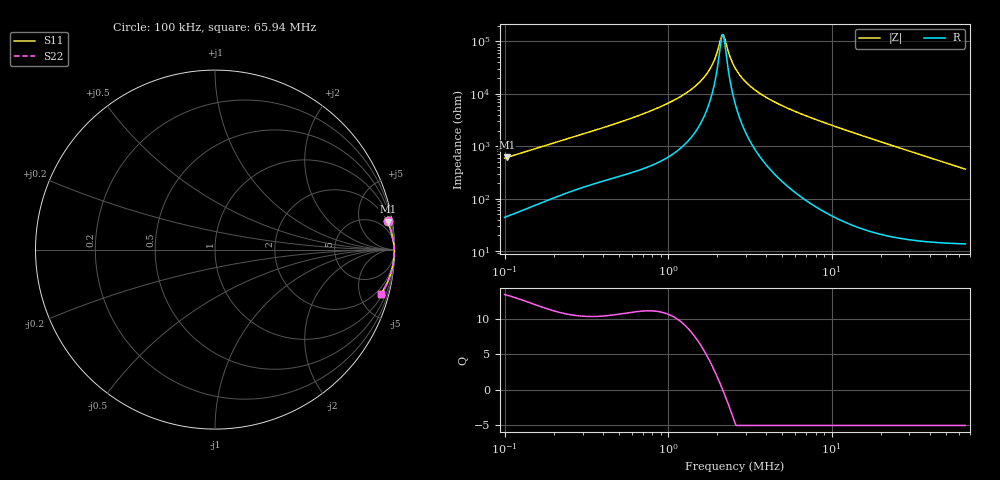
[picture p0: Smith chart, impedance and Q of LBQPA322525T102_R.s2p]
! LBQPA322525T102_R  S-PARAMETER MODEL  ( General Type )
! Model Generated by TAIYO YUDEN Corporation (http://www.ty-top.com)
! Version 1.0
! TAIYO YUDEN Control No. 191025NI43SB-FBB
! Copyright(c) 2019 TAIYO YUDEN CO.,LTD. All Rights Reserved.
! Product Description (link to TY-COMPAS)
! https://ds.yuden.co.jp/TYCOMPAS/or/detail?pn=LBQPA322525T102KR&u=M
! Products Name : Inductors
! Characteristics :
!  Inductance : 1000 uH , SRF(min) : 1.6 MHz , DC Resistance(max) : 16.9 Ohm
!  Rated Current : Saturation :100 mA , Temp Rise : 75 mA (20 degC)
!  Case Size : 3.2 x 2.5 / 0.126 x 0.098 [mm/inch] , Thickness : 2.5 / 0.098 [mm/inch]
!  (Conditions: Temperature = 25 degC , DC Bias Current/Voltage = 0A / 0V)
! External Node Assignments :
!  1  o---GGG---o  2
! GND o---------o GND
! Frequency Range : 0.1MHz  -  65.935307MHz  [ 402 STEP ]
# MHz S RI R 50
! Freq[MHz].  S11 Real  S11 Imag  S21 Real  S21 Imag  S12 Real  S12 Imag  S22 Real  S22 Imag
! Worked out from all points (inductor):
!   401 points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, 100 kHz to 65.94 MHz, reference 50 ohm
!   read as one part in series: L = 932 uH near 103.3 kHz
!   highest Q = 13.3 at 103.3 kHz (marker M1), where L = 941 uH
!   self-resonance near 2.148 MHz
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0.1  0.9612 0.1595  0.0388 -0.1595  0.0388 -0.1595  0.9612 0.1595
0.103299  0.963 0.1549  0.037 -0.1549  0.037 -0.1549  0.963 0.1549
0.296621  0.9909 0.0581  0.00906 -0.0581  0.00906 -0.0581  0.9909 0.0581
0.567694  0.9963 0.0304  0.00374 -0.0304  0.00374 -0.0304  0.9963 0.0304
0.879842  0.998 0.018  0.00196 -0.018  0.00196 -0.018  0.998 0.018
1.25735  0.9988 0.0101  0.0012 -0.0101  0.0012 -0.0101  0.9988 0.0101
1.431655  0.999 0.00753  0.00103 -0.00753  0.00103 -0.00753  0.999 0.00753
1.603884  0.9991 0.00539  0.000912 -0.00539  0.000912 -0.00539  0.9991 0.00539
1.73945  0.9992 0.0039  0.000846 -0.0039  0.000846 -0.0039  0.9992 0.0039
1.856107  0.9992 0.00272  0.000801 -0.00272  0.000801 -0.00272  0.9992 0.00272
1.948707  0.9992 0.00185  0.000773 -0.00185  0.000773 -0.00185  0.9992 0.00185
2.113418  0.9993 0.000397  0.000734 -0.000397  0.000734 -0.000397  0.9993 0.000397
2.147995  0.9993 0.000107  0.000727 -0.000107  0.000727 -0.000107  0.9993 0.000107
2.218855  0.9993 -0.000473  0.000715 0.000473  0.000715 0.000473  0.9993 -0.000473
2.4064  0.9993 -0.00193  0.000691 0.00193  0.000691 0.00193  0.9993 -0.00193
2.609798  0.9993 -0.00339  0.000676 0.00339  0.000676 0.00339  0.9993 -0.00339
3.020209  0.9993 -0.0061  0.000671 0.0061  0.000671 0.0061  0.9993 -0.0061
3.729566  0.9993 -0.0103  0.000713 0.0103  0.000713 0.0103  0.9993 -0.0103
4.994806  0.9991 -0.0168  0.000884 0.0168  0.000884 0.0168  0.9991 -0.0168
7.616602  0.9985 -0.029  0.0015 0.029  0.0015 0.029  0.9985 -0.029
22.59246  0.9898 -0.0918  0.0102 0.0918  0.0102 0.0918  0.9898 -0.0918
65.93531  0.9224 -0.2494  0.0776 0.2494  0.0776 0.2494  0.9224 -0.2494
